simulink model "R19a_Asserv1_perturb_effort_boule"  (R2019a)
settings: Solver=ode15s  StartTime=0.0  StopTime=1  RelTol=1e-3  EnableMultiTasking=on
undefined symbols (not defined in the file): deg, kg, m, manette1_Défaut_sldprt, manette2_Défaut_sldprt, mm, N, rad, s, sigbuilder_block, STL, X, Y, Z
libraries: sm_lib x460, fl_lib x45, nesl_utility x23, simulink x3
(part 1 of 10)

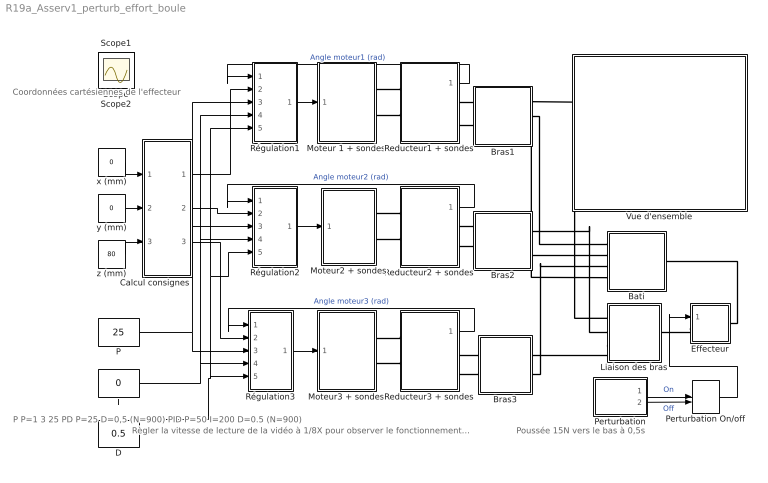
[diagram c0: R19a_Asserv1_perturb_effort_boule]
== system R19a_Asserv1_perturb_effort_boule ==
  note: P P=1 3 25 PD P=25 D=0,5 (N=900) PID P=50 I=200 D=0.5 (N=900)
  note: Coordonnées cartésiennes de l'effecteur
  note: Poussée 15N vers le bas à 0,5s
  note: Règler la vitesse de lecture de la vidéo à 1/8X pour observer le fonctionnement au ralenti
  Bati : Subsystem
  Bras1 : Subsystem
  Bras2 : Subsystem
  Bras3 : Subsystem
  Calcul consignes : Subsystem
  D : Constant  Value=0.5
  Effecteur : Subsystem
  I : Constant  Value=0
  Liaison des bras : Subsystem
  Moteur 1 + sondes : Subsystem
  Moteur2 + sondes : Subsystem
  Moteur3 + sondes : Subsystem
  P : Constant  Value=25
  Perturbation : Subsystem
  Perturbation On/off : ManualSwitch  CurrentSetting=0
  Reducteur1 + sondes : Subsystem
  Reducteur2 + sondes : Subsystem
  Reducteur3 + sondes : Subsystem
  Régulation1 : Subsystem
  Régulation2 : Subsystem
  Régulation3 : Subsystem
  Vue d'ensemble : Subsystem
  x (mm) : Constant  Value=0
  y (mm) : Constant  Value=0
  z (mm) : Constant  Value=80
  Scope : Scope
  Scope1 : Scope
  Scope2 : Scope
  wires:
  Régulation3/1(Out1) -> Moteur3 + sondes/1(In1)
  Reducteur3 + sondes/1(Angle_mot3) -> Régulation3/1(In1)  "Angle moteur3 (rad)"
  Régulation1/1(Out1) -> Moteur 1 + sondes/1(In1)
  Reducteur1 + sondes/1(Angle_mot1) -> Régulation1/1(In1)  "Angle moteur1 (rad)"
  Régulation2/1(Out1) -> Moteur2 + sondes/1(In1)
  Reducteur2 + sondes/1(Angle_mot2) -> Régulation2/1(In1)  "Angle moteur2 (rad)"
  Perturbation/1(Out1) -> Perturbation On/off/1  "On"
  Perturbation/2(Out2) -> Perturbation On/off/2  "Off"
  Perturbation On/off/1 -> Effecteur/1(In1)
  x (mm)/1 -> Calcul consignes/1(In1)
  y (mm)/1 -> Calcul consignes/2(In2)
  z (mm)/1 -> Calcul consignes/3(In3)
  Calcul consignes/1(C1) -> Régulation1/2(In2)
  Calcul consignes/2(C2) -> Régulation2/2(In2)
  Calcul consignes/3(C3) -> Régulation3/2(In2)
  P/1 -> Régulation3/3(P), Régulation1/3(P), Régulation2/3(P)
  I/1 -> Régulation1/4(I), Régulation2/4(I), Régulation3/4(I)
  D/1 -> Régulation1/5(D), Régulation2/5(D), Régulation3/5(D)
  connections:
  Moteur2 + sondes/RConn2 -- Reducteur2 + sondes/LConn2
  Moteur 1 + sondes/RConn1 -- Reducteur1 + sondes/LConn1
  Moteur3 + sondes/RConn2 -- Reducteur3 + sondes/LConn2
  Moteur2 + sondes/RConn1 -- Reducteur2 + sondes/LConn1
  Moteur3 + sondes/RConn1 -- Reducteur3 + sondes/LConn1
  Reducteur1 + sondes/LConn2 -- Moteur 1 + sondes/RConn2
  Bras1/LConn1 -- Reducteur1 + sondes/RConn1
  Reducteur1 + sondes/RConn2 -- Bras1/LConn2
  Bras2/LConn1 -- Reducteur2 + sondes/RConn1
  Bras2/LConn2 -- Reducteur2 + sondes/RConn2
  Reducteur3 + sondes/RConn1 -- Bras3/LConn1
  Reducteur3 + sondes/RConn2 -- Bras3/LConn2
  Bras1/RConn2 -- Bati/LConn1
  Bras2/RConn2 -- Bati/LConn2
  Bras3/RConn2 -- Bati/LConn3
  Liaison des bras/LConn1 -- Bras1/RConn1
  Liaison des bras/LConn2 -- Bras2/RConn1
  Effecteur/LConn1 -- Liaison des bras/RConn1
  Liaison des bras/LConn3 -- Bras3/RConn1
  Bati/RConn1 -- Effecteur/RConn1
  Bras1/RConn3 -- Bati/LConn4

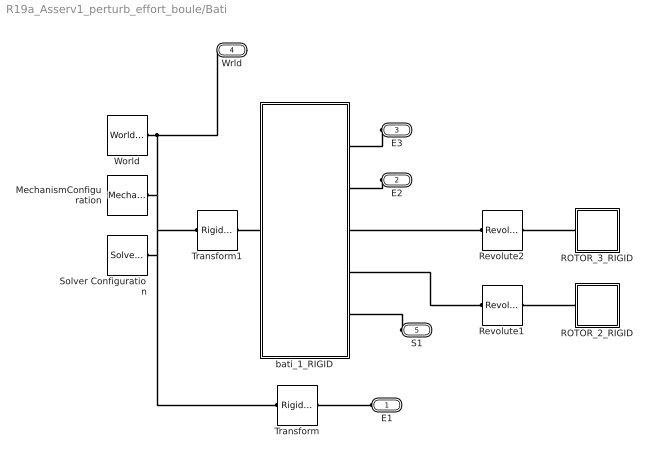
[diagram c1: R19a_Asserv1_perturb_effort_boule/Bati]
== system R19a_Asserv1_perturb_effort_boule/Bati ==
  MechanismConfiguration : sm_lib/Utilities/Mechanism Configuration  UniformGravity=Constant  GravityVector=[0 0 0]  GravityUnits=m/s^2  LinearizationDelta=0.001
  ROTOR_2_RIGID : Subsystem
  ROTOR_3_RIGID : Subsystem
  Revolute1 : sm_lib/Joints/Revolute Joint  SenseConstraintForce=off  SenseConstraintForceX=off  SenseConstraintForceY=off  SenseConstraintForceZ=off  SenseConstraintTorque=off  SenseConstraintTorqueX=off  SenseConstraintTorqueY=off  SenseConstraintTorqueZ=off  SenseTotalForce=off  SenseTotalForceX=off  SenseTotalForceY=off  SenseTotalForceZ=off  SenseTotalTorque=off  SenseTotalTorqueX=off  SenseTotalTorqueY=off  SenseTotalTorqueZ=off  CompositeWrenchDir=FollowerOnBase  CompositeWrenchFrame=BaseFrame  EquilibriumPosition=0  EquilibriumPositionUnits=rad  SpringStiffness=0  SpringStiffnessUnits=m*N/rad  DampingCoefficient=0  DampingCoefficientUnits=m*s*N/rad  TorqueActuationMode=NoTorque  MotionActuationMode=ComputedMotion  SensePosition=off  SenseVelocity=off  SenseAcceleration=off  SenseTorqueForce=off  SenseLowerLimitTorqueForce=off  SenseUpperLimitTorqueForce=off  LowerLimitSpecify=off  LowerLimitBound=-90  LowerLimitBoundUnits=deg  LowerLimitStiffness=1e4  LowerLimitStiffnessUnits=N*m/deg  LowerLimitDamping=10  LowerLimitDampingUnits=N*m/(deg/s)  LowerLimitTransitionRegionWidth=0.1  LowerLimitTransitionRegionWidthUnits=deg  UpperLimitSpecify=off  UpperLimitBound=90  UpperLimitBoundUnits=deg  UpperLimitStiffness=1e4  UpperLimitStiffnessUnits=N*m/deg  UpperLimitDamping=10  UpperLimitDampingUnits=N*m/(deg/s)  UpperLimitTransitionRegionWidth=0.1  UpperLimitTransitionRegionWidthUnits=deg  PositionTargetSpecify=on  PositionTargetPriority=Low  PositionTargetValue=-26.406351854743253  PositionTargetValueUnits=deg  VelocityTargetSpecify=off  VelocityTargetPriority=High  VelocityTargetValue=0  VelocityTargetValueUnits=deg/s
  Revolute2 : sm_lib/Joints/Revolute Joint  SenseConstraintForce=off  SenseConstraintForceX=off  SenseConstraintForceY=off  SenseConstraintForceZ=off  SenseConstraintTorque=off  SenseConstraintTorqueX=off  SenseConstraintTorqueY=off  SenseConstraintTorqueZ=off  SenseTotalForce=off  SenseTotalForceX=off  SenseTotalForceY=off  SenseTotalForceZ=off  SenseTotalTorque=off  SenseTotalTorqueX=off  SenseTotalTorqueY=off  SenseTotalTorqueZ=off  CompositeWrenchDir=FollowerOnBase  CompositeWrenchFrame=BaseFrame  EquilibriumPosition=0  EquilibriumPositionUnits=rad  SpringStiffness=0  SpringStiffnessUnits=m*N/rad  DampingCoefficient=0  DampingCoefficientUnits=m*s*N/rad  TorqueActuationMode=NoTorque  MotionActuationMode=ComputedMotion  SensePosition=off  SenseVelocity=off  SenseAcceleration=off  SenseTorqueForce=off  SenseLowerLimitTorqueForce=off  SenseUpperLimitTorqueForce=off  LowerLimitSpecify=off  LowerLimitBound=-90  LowerLimitBoundUnits=deg  LowerLimitStiffness=1e4  LowerLimitStiffnessUnits=N*m/deg  LowerLimitDamping=10  LowerLimitDampingUnits=N*m/(deg/s)  LowerLimitTransitionRegionWidth=0.1  LowerLimitTransitionRegionWidthUnits=deg  UpperLimitSpecify=off  UpperLimitBound=90  UpperLimitBoundUnits=deg  UpperLimitStiffness=1e4  UpperLimitStiffnessUnits=N*m/deg  UpperLimitDamping=10  UpperLimitDampingUnits=N*m/(deg/s)  UpperLimitTransitionRegionWidth=0.1  UpperLimitTransitionRegionWidthUnits=deg  PositionTargetSpecify=on  PositionTargetPriority=Low  PositionTargetValue=-61.713604489421797  PositionTargetValueUnits=deg  VelocityTargetSpecify=off  VelocityTargetPriority=High  VelocityTargetValue=0  VelocityTargetValueUnits=deg/s
  Solver Configuration : nesl_utility/Solver Configuration  PhysicalDomain=network_engine_domain  SubClassName=solver  LeftPortType=input  RightPortType=generic  Tones=[]  Harmonics=[]  SimulateNoise=off  Profile=off  UseLocalSampling=off  EnableSwitchedLinearOptims=on  FrequencyDomain=off  UseCCode=off  RelTol=0.001  AbsTol=1e-06  MinStep=1e-09  ToWorkspace=off  RevertToSquareIcSolve=off  NumHomotopyIterations=100  PhasorMode=off  PhasorModeNumHarmonics=1  DoDC=off  ResidualTolerance=1e-09  UseLocalSolver=off  LocalSolverChoice=NE_BACKWARD_EULER_ADVANCER  LocalSolverSampleTime=0.001  DoFixedCost=off  MaxNonlinIter=3  MaxModeIter=2  LinearAlgebra=Sparse  EquationFormulation=NE_TIME_EF  DelaysMemoryBudget=1024  AutomaticFiltering=on  FilteringTimeConstant=0.001  PartitionStorageMethod=AS_NEEDED  PartitionMemoryBudget=1024  PartitionMethod=FAST
  Transform : sm_lib/Frames and Transforms/Rigid Transform  TranslationMethod=Cartesian  TranslationStandardOffset=0  TranslationLengthUnit=mm  TranslationStandardAxis=+Z  TranslationCartesianOffset=[-50.295220189469383 24.641508789034031 0]  TranslationROffset=0  TranslationROffsetUnits=m  TranslationZOffset=0  TranslationZOffsetUnits=m  TranslationThetaOffset=0  TranslationThetaOffsetUnits=deg  RotationMethod=ArbitraryAxis  RotationAngleUnits=rad  RotationStandardAxis=+Z  RotationAngle=2.2576709855630148  RotationArbitraryAxis=[0.47317816576135285 0.62293756647304621 0.6229375664730461]  FollAlignAxisA=+X  BaseAlignAxisA=+Y  FollAlignAxisB=+Y  BaseAlignAxisB=+Z  RotationSequenceAxes=FollowerAxes  RotationSequence=XYX  RotationSequenceAngles=[0 0 0]  RotationSequenceAnglesUnits=deg  RotationMatrix=[1 0 0; 0 1 0; 0 0 1]
  Transform1 : sm_lib/Frames and Transforms/Rigid Transform  TranslationMethod=Cartesian  TranslationStandardOffset=0  TranslationLengthUnit=mm  TranslationStandardAxis=+Z  TranslationCartesianOffset=[0 -115.25004756062962 -99.318100969999989]  TranslationROffset=0  TranslationROffsetUnits=m  TranslationZOffset=0  TranslationZOffsetUnits=m  TranslationThetaOffset=0  TranslationThetaOffsetUnits=deg  RotationMethod=None  RotationAngleUnits=deg  RotationStandardAxis=+Z  RotationAngle=0  RotationArbitraryAxis=[0 0 1]  FollAlignAxisA=+X  BaseAlignAxisA=+Y  FollAlignAxisB=+Y  BaseAlignAxisB=+Z  RotationSequenceAxes=FollowerAxes  RotationSequence=XYX  RotationSequenceAngles=[0 0 0]  RotationSequenceAnglesUnits=deg  RotationMatrix=[1 0 0; 0 1 0; 0 0 1]
  World : sm_lib/Frames and Transforms/World Frame
  bati_1_RIGID : Subsystem
  E1 : PMIOPort  Side=Left
  E2 : PMIOPort  Port=2  Side=Left
  E3 : PMIOPort  Port=3  Side=Left
  Wrld : PMIOPort  Port=4  Side=Right
  S1 : PMIOPort  Port=5  Side=Left
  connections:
  MechanismConfiguration/RConn1 -- Transform/LConn1 -- Solver Configuration/RConn1 -- Transform1/LConn1 -- Wrld/RConn1 -- World/RConn1
  ROTOR_3_RIGID/LConn1 -- Revolute2/RConn1
  Transform1/RConn1 -- bati_1_RIGID/LConn1
  Revolute2/LConn1 -- bati_1_RIGID/RConn3
  E2/RConn1 -- bati_1_RIGID/RConn2
  E1/RConn1 -- Transform/RConn1
  E3/RConn1 -- bati_1_RIGID/RConn1
  ROTOR_2_RIGID/LConn1 -- Revolute1/RConn1
  S1/RConn1 -- bati_1_RIGID/RConn5
  Revolute1/LConn1 -- bati_1_RIGID/RConn4

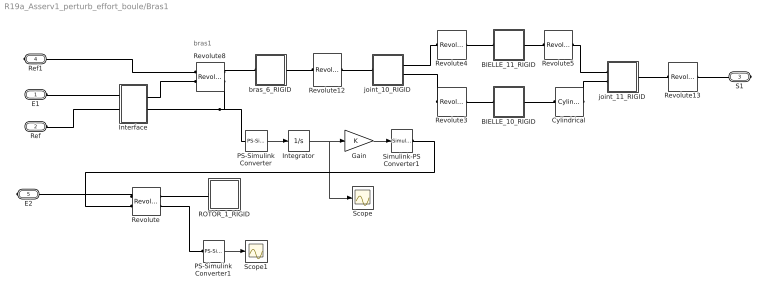
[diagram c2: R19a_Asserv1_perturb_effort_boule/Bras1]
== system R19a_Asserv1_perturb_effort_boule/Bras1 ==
  note: bras1
  BIELLE_10_RIGID : Subsystem
  BIELLE_11_RIGID : Subsystem
  Cylindrical : sm_lib/Joints/Cylindrical Joint  SenseConstraintForce=off  SenseConstraintForceX=off  SenseConstraintForceY=off  SenseConstraintForceZ=off  SenseConstraintTorque=off  SenseConstraintTorqueX=off  SenseConstraintTorqueY=off  SenseConstraintTorqueZ=off  SenseTotalForce=off  SenseTotalForceX=off  SenseTotalForceY=off  SenseTotalForceZ=off  SenseTotalTorque=off  SenseTotalTorqueX=off  SenseTotalTorqueY=off  SenseTotalTorqueZ=off  CompositeWrenchDir=FollowerOnBase  CompositeWrenchFrame=BaseFrame  PzEquilibriumPosition=0  PzEquilibriumPositionUnits=m  PzSpringStiffness=0  PzSpringStiffnessUnits=N/m  PzDampingCoefficient=0  PzDampingCoefficientUnits=s*N/m  PzTorqueActuationMode=NoTorque  PzMotionActuationMode=ComputedMotion  PzSensePosition=off  PzSenseVelocity=off  PzSenseAcceleration=off  PzSenseTorqueForce=off  PzSenseLowerLimitTorqueForce=off  PzSenseUpperLimitTorqueForce=off  PzLowerLimitSpecify=off  PzLowerLimitBound=-1  PzLowerLimitBoundUnits=m  PzLowerLimitStiffness=1e6  PzLowerLimitStiffnessUnits=N/m  PzLowerLimitDamping=1e3  PzLowerLimitDampingUnits=N/(m/s)  PzLowerLimitTransitionRegionWidth=1e-4  PzLowerLimitTransitionRegionWidthUnits=m  PzUpperLimitSpecify=off  PzUpperLimitBound=1  PzUpperLimitBoundUnits=m  PzUpperLimitStiffness=1e6  PzUpperLimitStiffnessUnits=N/m  PzUpperLimitDamping=1e3  PzUpperLimitDampingUnits=N/(m/s)  PzUpperLimitTransitionRegionWidth=1e-4  PzUpperLimitTransitionRegionWidthUnits=m  PzPositionTargetSpecify=off  PzPositionTargetPriority=High  PzPositionTargetValue=0  PzPositionTargetValueUnits=m  PzVelocityTargetSpecify=off  PzVelocityTargetPriority=High  PzVelocityTargetValue=0  PzVelocityTargetValueUnits=m/s  RzEquilibriumPosition=0  RzEquilibriumPositionUnits=rad  RzSpringStiffness=0  RzSpringStiffnessUnits=m*N/rad  RzDampingCoefficient=0  RzDampingCoefficientUnits=m*s*N/rad  RzTorqueActuationMode=NoTorque  RzMotionActuationMode=ComputedMotion  RzSensePosition=off  RzSenseVelocity=off  RzSenseAcceleration=off  RzSenseTorqueForce=off  RzSenseLowerLimitTorqueForce=off  RzSenseUpperLimitTorqueForce=off  RzLowerLimitSpecify=off  RzLowerLimitBound=-90  RzLowerLimitBoundUnits=deg  RzLowerLimitStiffness=1e4  RzLowerLimitStiffnessUnits=N*m/deg  RzLowerLimitDamping=10  RzLowerLimitDampingUnits=N*m/(deg/s)  RzLowerLimitTransitionRegionWidth=0.1  RzLowerLimitTransitionRegionWidthUnits=deg  RzUpperLimitSpecify=off  RzUpperLimitBound=90  RzUpperLimitBoundUnits=deg  RzUpperLimitStiffness=1e4  RzUpperLimitStiffnessUnits=N*m/deg  RzUpperLimitDamping=10  RzUpperLimitDampingUnits=N*m/(deg/s)  RzUpperLimitTransitionRegionWidth=0.1  RzUpperLimitTransitionRegionWidthUnits=deg  RzPositionTargetSpecify=off  RzPositionTargetPriority=High  RzPositionTargetValue=0  RzPositionTargetValueUnits=deg  RzVelocityTargetSpecify=off  RzVelocityTargetPriority=High  RzVelocityTargetValue=0  RzVelocityTargetValueUnits=deg/s
  Gain : Gain
  Integrator : Integrator
  Interface : Subsystem
  PS-Simulink Converter : nesl_utility/PS-Simulink Converter  PhysicalDomain=network_engine_domain  SubClassName=ps_output  LeftPortType=input  RightPortType=output  PseudoPeriodic=off  Frequencies=[]  Unit=1  AffineConversion=off
  PS-Simulink Converter1 : nesl_utility/PS-Simulink Converter  PhysicalDomain=network_engine_domain  SubClassName=ps_output  LeftPortType=input  RightPortType=output  PseudoPeriodic=off  Frequencies=[]  Unit=1  AffineConversion=off
  ROTOR_1_RIGID : Subsystem
  Revolute : sm_lib/Joints/Revolute Joint  SenseConstraintForce=off  SenseConstraintForceX=off  SenseConstraintForceY=off  SenseConstraintForceZ=off  SenseConstraintTorque=off  SenseConstraintTorqueX=off  SenseConstraintTorqueY=off  SenseConstraintTorqueZ=off  SenseTotalForce=off  SenseTotalForceX=off  SenseTotalForceY=off  SenseTotalForceZ=off  SenseTotalTorque=off  SenseTotalTorqueX=off  SenseTotalTorqueY=off  SenseTotalTorqueZ=off  CompositeWrenchDir=FollowerOnBase  CompositeWrenchFrame=BaseFrame  EquilibriumPosition=0  EquilibriumPositionUnits=rad  SpringStiffness=0  SpringStiffnessUnits=m*N/rad  DampingCoefficient=0  DampingCoefficientUnits=m*s*N/rad  TorqueActuationMode=ComputedTorque  MotionActuationMode=InputMotion  SensePosition=off  SenseVelocity=on  SenseAcceleration=off  SenseTorqueForce=off  SenseLowerLimitTorqueForce=off  SenseUpperLimitTorqueForce=off  LowerLimitSpecify=off  LowerLimitBound=-90  LowerLimitBoundUnits=deg  LowerLimitStiffness=1e4  LowerLimitStiffnessUnits=N*m/deg  LowerLimitDamping=10  LowerLimitDampingUnits=N*m/(deg/s)  LowerLimitTransitionRegionWidth=0.1  LowerLimitTransitionRegionWidthUnits=deg  UpperLimitSpecify=off  UpperLimitBound=90  UpperLimitBoundUnits=deg  UpperLimitStiffness=1e4  UpperLimitStiffnessUnits=N*m/deg  UpperLimitDamping=10  UpperLimitDampingUnits=N*m/(deg/s)  UpperLimitTransitionRegionWidth=0.1  UpperLimitTransitionRegionWidthUnits=deg  PositionTargetSpecify=on  PositionTargetPriority=Low  PositionTargetValue=-79.560971310790379  PositionTargetValueUnits=deg  VelocityTargetSpecify=off  VelocityTargetPriority=High  VelocityTargetValue=0  VelocityTargetValueUnits=deg/s
  Revolute12 : sm_lib/Joints/Revolute Joint  SenseConstraintForce=off  SenseConstraintForceX=off  SenseConstraintForceY=off  SenseConstraintForceZ=off  SenseConstraintTorque=off  SenseConstraintTorqueX=off  SenseConstraintTorqueY=off  SenseConstraintTorqueZ=off  SenseTotalForce=off  SenseTotalForceX=off  SenseTotalForceY=off  SenseTotalForceZ=off  SenseTotalTorque=off  SenseTotalTorqueX=off  SenseTotalTorqueY=off  SenseTotalTorqueZ=off  CompositeWrenchDir=FollowerOnBase  CompositeWrenchFrame=BaseFrame  EquilibriumPosition=0  EquilibriumPositionUnits=rad  SpringStiffness=0  SpringStiffnessUnits=m*N/rad  DampingCoefficient=0  DampingCoefficientUnits=m*s*N/rad  TorqueActuationMode=NoTorque  MotionActuationMode=ComputedMotion  SensePosition=off  SenseVelocity=off  SenseAcceleration=off  SenseTorqueForce=off  SenseLowerLimitTorqueForce=off  SenseUpperLimitTorqueForce=off  LowerLimitSpecify=off  LowerLimitBound=-90  LowerLimitBoundUnits=deg  LowerLimitStiffness=1e4  LowerLimitStiffnessUnits=N*m/deg  LowerLimitDamping=10  LowerLimitDampingUnits=N*m/(deg/s)  LowerLimitTransitionRegionWidth=0.1  LowerLimitTransitionRegionWidthUnits=deg  UpperLimitSpecify=off  UpperLimitBound=90  UpperLimitBoundUnits=deg  UpperLimitStiffness=1e4  UpperLimitStiffnessUnits=N*m/deg  UpperLimitDamping=10  UpperLimitDampingUnits=N*m/(deg/s)  UpperLimitTransitionRegionWidth=0.1  UpperLimitTransitionRegionWidthUnits=deg  PositionTargetSpecify=on  PositionTargetPriority=Low  PositionTargetValue=114.87234196171698  PositionTargetValueUnits=deg  VelocityTargetSpecify=off  VelocityTargetPriority=High  VelocityTargetValue=0  VelocityTargetValueUnits=deg/s
  Revolute13 : sm_lib/Joints/Revolute Joint  SenseConstraintForce=off  SenseConstraintForceX=off  SenseConstraintForceY=off  SenseConstraintForceZ=off  SenseConstraintTorque=off  SenseConstraintTorqueX=off  SenseConstraintTorqueY=off  SenseConstraintTorqueZ=off  SenseTotalForce=off  SenseTotalForceX=off  SenseTotalForceY=off  SenseTotalForceZ=off  SenseTotalTorque=off  SenseTotalTorqueX=off  SenseTotalTorqueY=off  SenseTotalTorqueZ=off  CompositeWrenchDir=FollowerOnBase  CompositeWrenchFrame=BaseFrame  EquilibriumPosition=0  EquilibriumPositionUnits=rad  SpringStiffness=0  SpringStiffnessUnits=m*N/rad  DampingCoefficient=0  DampingCoefficientUnits=m*s*N/rad  TorqueActuationMode=NoTorque  MotionActuationMode=ComputedMotion  SensePosition=off  SenseVelocity=off  SenseAcceleration=off  SenseTorqueForce=off  SenseLowerLimitTorqueForce=off  SenseUpperLimitTorqueForce=off  LowerLimitSpecify=off  LowerLimitBound=-90  LowerLimitBoundUnits=deg  LowerLimitStiffness=1e4  LowerLimitStiffnessUnits=N*m/deg  LowerLimitDamping=10  LowerLimitDampingUnits=N*m/(deg/s)  LowerLimitTransitionRegionWidth=0.1  LowerLimitTransitionRegionWidthUnits=deg  UpperLimitSpecify=off  UpperLimitBound=90  UpperLimitBoundUnits=deg  UpperLimitStiffness=1e4  UpperLimitStiffnessUnits=N*m/deg  UpperLimitDamping=10  UpperLimitDampingUnits=N*m/(deg/s)  UpperLimitTransitionRegionWidth=0.1  UpperLimitTransitionRegionWidthUnits=deg  PositionTargetSpecify=off  PositionTargetPriority=High  PositionTargetValue=0  PositionTargetValueUnits=deg  VelocityTargetSpecify=off  VelocityTargetPriority=High  VelocityTargetValue=0  VelocityTargetValueUnits=deg/s
  Revolute3 : sm_lib/Joints/Revolute Joint  SenseConstraintForce=off  SenseConstraintForceX=off  SenseConstraintForceY=off  SenseConstraintForceZ=off  SenseConstraintTorque=off  SenseConstraintTorqueX=off  SenseConstraintTorqueY=off  SenseConstraintTorqueZ=off  SenseTotalForce=off  SenseTotalForceX=off  SenseTotalForceY=off  SenseTotalForceZ=off  SenseTotalTorque=off  SenseTotalTorqueX=off  SenseTotalTorqueY=off  SenseTotalTorqueZ=off  CompositeWrenchDir=FollowerOnBase  CompositeWrenchFrame=BaseFrame  EquilibriumPosition=0  EquilibriumPositionUnits=rad  SpringStiffness=0  SpringStiffnessUnits=m*N/rad  DampingCoefficient=0  DampingCoefficientUnits=m*s*N/rad  TorqueActuationMode=NoTorque  MotionActuationMode=ComputedMotion  SensePosition=off  SenseVelocity=off  SenseAcceleration=off  SenseTorqueForce=off  SenseLowerLimitTorqueForce=off  SenseUpperLimitTorqueForce=off  LowerLimitSpecify=off  LowerLimitBound=-90  LowerLimitBoundUnits=deg  LowerLimitStiffness=1e4  LowerLimitStiffnessUnits=N*m/deg  LowerLimitDamping=10  LowerLimitDampingUnits=N*m/(deg/s)  LowerLimitTransitionRegionWidth=0.1  LowerLimitTransitionRegionWidthUnits=deg  UpperLimitSpecify=off  UpperLimitBound=90  UpperLimitBoundUnits=deg  UpperLimitStiffness=1e4  UpperLimitStiffnessUnits=N*m/deg  UpperLimitDamping=10  UpperLimitDampingUnits=N*m/(deg/s)  UpperLimitTransitionRegionWidth=0.1  UpperLimitTransitionRegionWidthUnits=deg  PositionTargetSpecify=on  PositionTargetPriority=Low  PositionTargetValue=-1.4448284825041595  PositionTargetValueUnits=deg  VelocityTargetSpecify=off  VelocityTargetPriority=High  VelocityTargetValue=0  VelocityTargetValueUnits=deg/s
  Revolute4 : sm_lib/Joints/Revolute Joint  SenseConstraintForce=off  SenseConstraintForceX=off  SenseConstraintForceY=off  SenseConstraintForceZ=off  SenseConstraintTorque=off  SenseConstraintTorqueX=off  SenseConstraintTorqueY=off  SenseConstraintTorqueZ=off  SenseTotalForce=off  SenseTotalForceX=off  SenseTotalForceY=off  SenseTotalForceZ=off  SenseTotalTorque=off  SenseTotalTorqueX=off  SenseTotalTorqueY=off  SenseTotalTorqueZ=off  CompositeWrenchDir=FollowerOnBase  CompositeWrenchFrame=BaseFrame  EquilibriumPosition=0  EquilibriumPositionUnits=rad  SpringStiffness=0  SpringStiffnessUnits=m*N/rad  DampingCoefficient=0  DampingCoefficientUnits=m*s*N/rad  TorqueActuationMode=NoTorque  MotionActuationMode=ComputedMotion  SensePosition=off  SenseVelocity=off  SenseAcceleration=off  SenseTorqueForce=off  SenseLowerLimitTorqueForce=off  SenseUpperLimitTorqueForce=off  LowerLimitSpecify=off  LowerLimitBound=-90  LowerLimitBoundUnits=deg  LowerLimitStiffness=1e4  LowerLimitStiffnessUnits=N*m/deg  LowerLimitDamping=10  LowerLimitDampingUnits=N*m/(deg/s)  LowerLimitTransitionRegionWidth=0.1  LowerLimitTransitionRegionWidthUnits=deg  UpperLimitSpecify=off  UpperLimitBound=90  UpperLimitBoundUnits=deg  UpperLimitStiffness=1e4  UpperLimitStiffnessUnits=N*m/deg  UpperLimitDamping=10  UpperLimitDampingUnits=N*m/(deg/s)  UpperLimitTransitionRegionWidth=0.1  UpperLimitTransitionRegionWidthUnits=deg  PositionTargetSpecify=on  PositionTargetPriority=Low  PositionTargetValue=1.4448284825041535  PositionTargetValueUnits=deg  VelocityTargetSpecify=off  VelocityTargetPriority=High  VelocityTargetValue=0  VelocityTargetValueUnits=deg/s
  Revolute5 : sm_lib/Joints/Revolute Joint  SenseConstraintForce=off  SenseConstraintForceX=off  SenseConstraintForceY=off  SenseConstraintForceZ=off  SenseConstraintTorque=off  SenseConstraintTorqueX=off  SenseConstraintTorqueY=off  SenseConstraintTorqueZ=off  SenseTotalForce=off  SenseTotalForceX=off  SenseTotalForceY=off  SenseTotalForceZ=off  SenseTotalTorque=off  SenseTotalTorqueX=off  SenseTotalTorqueY=off  SenseTotalTorqueZ=off  CompositeWrenchDir=FollowerOnBase  CompositeWrenchFrame=BaseFrame  EquilibriumPosition=0  EquilibriumPositionUnits=rad  SpringStiffness=0  SpringStiffnessUnits=m*N/rad  DampingCoefficient=0  DampingCoefficientUnits=m*s*N/rad  TorqueActuationMode=NoTorque  MotionActuationMode=ComputedMotion  SensePosition=off  SenseVelocity=off  SenseAcceleration=off  SenseTorqueForce=off  SenseLowerLimitTorqueForce=off  SenseUpperLimitTorqueForce=off  LowerLimitSpecify=off  LowerLimitBound=-90  LowerLimitBoundUnits=deg  LowerLimitStiffness=1e4  LowerLimitStiffnessUnits=N*m/deg  LowerLimitDamping=10  LowerLimitDampingUnits=N*m/(deg/s)  LowerLimitTransitionRegionWidth=0.1  LowerLimitTransitionRegionWidthUnits=deg  UpperLimitSpecify=off  UpperLimitBound=90  UpperLimitBoundUnits=deg  UpperLimitStiffness=1e4  UpperLimitStiffnessUnits=N*m/deg  UpperLimitDamping=10  UpperLimitDampingUnits=N*m/(deg/s)  UpperLimitTransitionRegionWidth=0.1  UpperLimitTransitionRegionWidthUnits=deg  PositionTargetSpecify=on  PositionTargetPriority=Low  PositionTargetValue=-178.55517151749589  PositionTargetValueUnits=deg  VelocityTargetSpecify=off  VelocityTargetPriority=High  VelocityTargetValue=0  VelocityTargetValueUnits=deg/s
  Revolute8 : sm_lib/Joints/Revolute Joint  SenseConstraintForce=off  SenseConstraintForceX=off  SenseConstraintForceY=off  SenseConstraintForceZ=off  SenseConstraintTorque=off  SenseConstraintTorqueX=off  SenseConstraintTorqueY=off  SenseConstraintTorqueZ=off  SenseTotalForce=off  SenseTotalForceX=off  SenseTotalForceY=off  SenseTotalForceZ=off  SenseTotalTorque=off  SenseTotalTorqueX=off  SenseTotalTorqueY=off  SenseTotalTorqueZ=off  CompositeWrenchDir=FollowerOnBase  CompositeWrenchFrame=BaseFrame  EquilibriumPosition=0  EquilibriumPositionUnits=rad  SpringStiffness=0  SpringStiffnessUnits=m*N/rad  DampingCoefficient=0  DampingCoefficientUnits=m*s*N/rad  TorqueActuationMode=InputTorque  MotionActuationMode=ComputedMotion  SensePosition=off  SenseVelocity=on  SenseAcceleration=off  SenseTorqueForce=off  SenseLowerLimitTorqueForce=off  SenseUpperLimitTorqueForce=off  LowerLimitSpecify=off  LowerLimitBound=-90  LowerLimitBoundUnits=deg  LowerLimitStiffness=1e4  LowerLimitStiffnessUnits=N*m/deg  LowerLimitDamping=10  LowerLimitDampingUnits=N*m/(deg/s)  LowerLimitTransitionRegionWidth=0.1  LowerLimitTransitionRegionWidthUnits=deg  UpperLimitSpecify=off  UpperLimitBound=90  UpperLimitBoundUnits=deg  UpperLimitStiffness=1e4  UpperLimitStiffnessUnits=N*m/deg  UpperLimitDamping=10  UpperLimitDampingUnits=N*m/(deg/s)  UpperLimitTransitionRegionWidth=0.1  UpperLimitTransitionRegionWidthUnits=deg  PositionTargetSpecify=on  PositionTargetPriority=Low  PositionTargetValue=-11.877849818911594  PositionTargetValueUnits=deg  VelocityTargetSpecify=off  VelocityTargetPriority=High  VelocityTargetValue=0  VelocityTargetValueUnits=deg/s
  Scope : Scope
  Scope1 : Scope
  Simulink-PS Converter1 : nesl_utility/Simulink-PS Converter  PhysicalDomain=network_engine_domain  SubClassName=ps_input  LeftPortType=input  RightPortType=output  PseudoPeriodic=off  Frequencies=[]  NoiseDistribution=none  NoiseParameters=[]  Unit=1  AffineConversion=off  FilteringAndDerivatives=filter  SimscapeFilterOrder=2  InputFilterTimeConstant=1e-4  UdotUserProvided=1
  bras_6_RIGID : Subsystem
  joint_10_RIGID : Subsystem
  joint_11_RIGID : Subsystem
  E1 : PMIOPort  Side=Left
  Ref : PMIOPort  Port=2  Side=Left
  S1 : PMIOPort  Port=3  Side=Right
  Ref1 : PMIOPort  Port=4  Side=Right
  E2 : PMIOPort  Port=5  Side=Right
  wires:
  PS-Simulink Converter/1 -> Integrator/1
  Gain/1 -> Simulink-PS Converter1/1
  PS-Simulink Converter1/1 -> Scope1/1
  Integrator/1 -> Scope/1, Gain/1
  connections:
  Interface/RConn1 -- Revolute8/LConn2
  Interface/RConn2 -- PS-Simulink Converter/LConn1 -- Revolute8/RConn2
  Ref/RConn1 -- Interface/LConn2
  Interface/LConn1 -- E1/RConn1
  BIELLE_11_RIGID/LConn1 -- Revolute4/LConn1
  BIELLE_10_RIGID/RConn1 -- Cylindrical/LConn1
  Revolute4/RConn1 -- joint_10_RIGID/RConn1
  Cylindrical/RConn1 -- joint_11_RIGID/LConn2
  BIELLE_11_RIGID/RConn1 -- Revolute5/LConn1
  Revolute12/LConn1 -- bras_6_RIGID/RConn1
  Revolute12/RConn1 -- joint_10_RIGID/LConn1
  Revolute8/RConn1 -- bras_6_RIGID/LConn1
  Revolute8/LConn1 -- Ref1/RConn1
  Revolute5/RConn1 -- joint_11_RIGID/LConn1
  Revolute13/RConn1 -- joint_11_RIGID/RConn1
  S1/RConn1 -- Revolute13/LConn1
  Revolute3/RConn1 -- joint_10_RIGID/RConn2
  BIELLE_10_RIGID/LConn1 -- Revolute3/LConn1
  ROTOR_1_RIGID/LConn1 -- Revolute/RConn1
  Revolute/LConn1 -- E2/RConn1
  Revolute/LConn2 -- Simulink-PS Converter1/RConn1
  PS-Simulink Converter1/LConn1 -- Revolute/RConn2

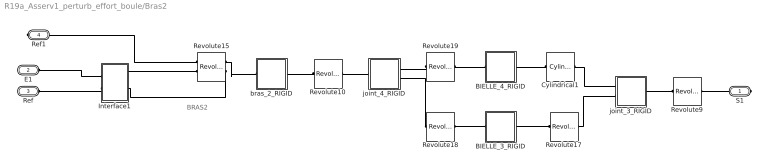
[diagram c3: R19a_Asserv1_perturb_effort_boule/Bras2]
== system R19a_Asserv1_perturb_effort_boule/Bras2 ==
  note: BRAS2
  BIELLE_3_RIGID : Subsystem
  BIELLE_4_RIGID : Subsystem
  Cylindrical1 : sm_lib/Joints/Cylindrical Joint  SenseConstraintForce=off  SenseConstraintForceX=off  SenseConstraintForceY=off  SenseConstraintForceZ=off  SenseConstraintTorque=off  SenseConstraintTorqueX=off  SenseConstraintTorqueY=off  SenseConstraintTorqueZ=off  SenseTotalForce=off  SenseTotalForceX=off  SenseTotalForceY=off  SenseTotalForceZ=off  SenseTotalTorque=off  SenseTotalTorqueX=off  SenseTotalTorqueY=off  SenseTotalTorqueZ=off  CompositeWrenchDir=FollowerOnBase  CompositeWrenchFrame=BaseFrame  PzEquilibriumPosition=0  PzEquilibriumPositionUnits=m  PzSpringStiffness=0  PzSpringStiffnessUnits=N/m  PzDampingCoefficient=0  PzDampingCoefficientUnits=s*N/m  PzTorqueActuationMode=NoTorque  PzMotionActuationMode=ComputedMotion  PzSensePosition=off  PzSenseVelocity=off  PzSenseAcceleration=off  PzSenseTorqueForce=off  PzSenseLowerLimitTorqueForce=off  PzSenseUpperLimitTorqueForce=off  PzLowerLimitSpecify=off  PzLowerLimitBound=-1  PzLowerLimitBoundUnits=m  PzLowerLimitStiffness=1e6  PzLowerLimitStiffnessUnits=N/m  PzLowerLimitDamping=1e3  PzLowerLimitDampingUnits=N/(m/s)  PzLowerLimitTransitionRegionWidth=1e-4  PzLowerLimitTransitionRegionWidthUnits=m  PzUpperLimitSpecify=off  PzUpperLimitBound=1  PzUpperLimitBoundUnits=m  PzUpperLimitStiffness=1e6  PzUpperLimitStiffnessUnits=N/m  PzUpperLimitDamping=1e3  PzUpperLimitDampingUnits=N/(m/s)  PzUpperLimitTransitionRegionWidth=1e-4  PzUpperLimitTransitionRegionWidthUnits=m  PzPositionTargetSpecify=off  PzPositionTargetPriority=High  PzPositionTargetValue=0  PzPositionTargetValueUnits=m  PzVelocityTargetSpecify=off  PzVelocityTargetPriority=High  PzVelocityTargetValue=0  PzVelocityTargetValueUnits=m/s  RzEquilibriumPosition=0  RzEquilibriumPositionUnits=rad  RzSpringStiffness=0  RzSpringStiffnessUnits=m*N/rad  RzDampingCoefficient=0  RzDampingCoefficientUnits=m*s*N/rad  RzTorqueActuationMode=NoTorque  RzMotionActuationMode=ComputedMotion  RzSensePosition=off  RzSenseVelocity=off  RzSenseAcceleration=off  RzSenseTorqueForce=off  RzSenseLowerLimitTorqueForce=off  RzSenseUpperLimitTorqueForce=off  RzLowerLimitSpecify=off  RzLowerLimitBound=-90  RzLowerLimitBoundUnits=deg  RzLowerLimitStiffness=1e4  RzLowerLimitStiffnessUnits=N*m/deg  RzLowerLimitDamping=10  RzLowerLimitDampingUnits=N*m/(deg/s)  RzLowerLimitTransitionRegionWidth=0.1  RzLowerLimitTransitionRegionWidthUnits=deg  RzUpperLimitSpecify=off  RzUpperLimitBound=90  RzUpperLimitBoundUnits=deg  RzUpperLimitStiffness=1e4  RzUpperLimitStiffnessUnits=N*m/deg  RzUpperLimitDamping=10  RzUpperLimitDampingUnits=N*m/(deg/s)  RzUpperLimitTransitionRegionWidth=0.1  RzUpperLimitTransitionRegionWidthUnits=deg  RzPositionTargetSpecify=off  RzPositionTargetPriority=High  RzPositionTargetValue=0  RzPositionTargetValueUnits=deg  RzVelocityTargetSpecify=off  RzVelocityTargetPriority=High  RzVelocityTargetValue=0  RzVelocityTargetValueUnits=deg/s
  Interface1 : Subsystem
  Revolute10 : sm_lib/Joints/Revolute Joint  SenseConstraintForce=off  SenseConstraintForceX=off  SenseConstraintForceY=off  SenseConstraintForceZ=off  SenseConstraintTorque=off  SenseConstraintTorqueX=off  SenseConstraintTorqueY=off  SenseConstraintTorqueZ=off  SenseTotalForce=off  SenseTotalForceX=off  SenseTotalForceY=off  SenseTotalForceZ=off  SenseTotalTorque=off  SenseTotalTorqueX=off  SenseTotalTorqueY=off  SenseTotalTorqueZ=off  CompositeWrenchDir=FollowerOnBase  CompositeWrenchFrame=BaseFrame  EquilibriumPosition=0  EquilibriumPositionUnits=rad  SpringStiffness=0  SpringStiffnessUnits=m*N/rad  DampingCoefficient=0  DampingCoefficientUnits=m*s*N/rad  TorqueActuationMode=NoTorque  MotionActuationMode=ComputedMotion  SensePosition=off  SenseVelocity=off  SenseAcceleration=off  SenseTorqueForce=off  SenseLowerLimitTorqueForce=off  SenseUpperLimitTorqueForce=off  LowerLimitSpecify=off  LowerLimitBound=-90  LowerLimitBoundUnits=deg  LowerLimitStiffness=1e4  LowerLimitStiffnessUnits=N*m/deg  LowerLimitDamping=10  LowerLimitDampingUnits=N*m/(deg/s)  LowerLimitTransitionRegionWidth=0.1  LowerLimitTransitionRegionWidthUnits=deg  UpperLimitSpecify=off  UpperLimitBound=90  UpperLimitBoundUnits=deg  UpperLimitStiffness=1e4  UpperLimitStiffnessUnits=N*m/deg  UpperLimitDamping=10  UpperLimitDampingUnits=N*m/(deg/s)  UpperLimitTransitionRegionWidth=0.1  UpperLimitTransitionRegionWidthUnits=deg  PositionTargetSpecify=on  PositionTargetPriority=Low  PositionTargetValue=114.872364906431  PositionTargetValueUnits=deg  VelocityTargetSpecify=off  VelocityTargetPriority=High  VelocityTargetValue=0  VelocityTargetValueUnits=deg/s
  Revolute15 : sm_lib/Joints/Revolute Joint  SenseConstraintForce=off  SenseConstraintForceX=off  SenseConstraintForceY=off  SenseConstraintForceZ=off  SenseConstraintTorque=off  SenseConstraintTorqueX=off  SenseConstraintTorqueY=off  SenseConstraintTorqueZ=off  SenseTotalForce=off  SenseTotalForceX=off  SenseTotalForceY=off  SenseTotalForceZ=off  SenseTotalTorque=off  SenseTotalTorqueX=off  SenseTotalTorqueY=off  SenseTotalTorqueZ=off  CompositeWrenchDir=FollowerOnBase  CompositeWrenchFrame=BaseFrame  EquilibriumPosition=0  EquilibriumPositionUnits=rad  SpringStiffness=0  SpringStiffnessUnits=m*N/rad  DampingCoefficient=0  DampingCoefficientUnits=m*s*N/rad  TorqueActuationMode=InputTorque  MotionActuationMode=ComputedMotion  SensePosition=off  SenseVelocity=on  SenseAcceleration=off  SenseTorqueForce=off  SenseLowerLimitTorqueForce=off  SenseUpperLimitTorqueForce=off  LowerLimitSpecify=off  LowerLimitBound=-90  LowerLimitBoundUnits=deg  LowerLimitStiffness=1e4  LowerLimitStiffnessUnits=N*m/deg  LowerLimitDamping=10  LowerLimitDampingUnits=N*m/(deg/s)  LowerLimitTransitionRegionWidth=0.1  LowerLimitTransitionRegionWidthUnits=deg  UpperLimitSpecify=off  UpperLimitBound=90  UpperLimitBoundUnits=deg  UpperLimitStiffness=1e4  UpperLimitStiffnessUnits=N*m/deg  UpperLimitDamping=10  UpperLimitDampingUnits=N*m/(deg/s)  UpperLimitTransitionRegionWidth=0.1  UpperLimitTransitionRegionWidthUnits=deg  PositionTargetSpecify=on  PositionTargetPriority=Low  PositionTargetValue=-168.12223208512529  PositionTargetValueUnits=deg  VelocityTargetSpecify=off  VelocityTargetPriority=High  VelocityTargetValue=0  VelocityTargetValueUnits=deg/s
  Revolute17 : sm_lib/Joints/Revolute Joint  SenseConstraintForce=off  SenseConstraintForceX=off  SenseConstraintForceY=off  SenseConstraintForceZ=off  SenseConstraintTorque=off  SenseConstraintTorqueX=off  SenseConstraintTorqueY=off  SenseConstraintTorqueZ=off  SenseTotalForce=off  SenseTotalForceX=off  SenseTotalForceY=off  SenseTotalForceZ=off  SenseTotalTorque=off  SenseTotalTorqueX=off  SenseTotalTorqueY=off  SenseTotalTorqueZ=off  CompositeWrenchDir=FollowerOnBase  CompositeWrenchFrame=BaseFrame  EquilibriumPosition=0  EquilibriumPositionUnits=rad  SpringStiffness=0  SpringStiffnessUnits=m*N/rad  DampingCoefficient=0  DampingCoefficientUnits=m*s*N/rad  TorqueActuationMode=NoTorque  MotionActuationMode=ComputedMotion  SensePosition=off  SenseVelocity=off  SenseAcceleration=off  SenseTorqueForce=off  SenseLowerLimitTorqueForce=off  SenseUpperLimitTorqueForce=off  LowerLimitSpecify=off  LowerLimitBound=-90  LowerLimitBoundUnits=deg  LowerLimitStiffness=1e4  LowerLimitStiffnessUnits=N*m/deg  LowerLimitDamping=10  LowerLimitDampingUnits=N*m/(deg/s)  LowerLimitTransitionRegionWidth=0.1  LowerLimitTransitionRegionWidthUnits=deg  UpperLimitSpecify=off  UpperLimitBound=90  UpperLimitBoundUnits=deg  UpperLimitStiffness=1e4  UpperLimitStiffnessUnits=N*m/deg  UpperLimitDamping=10  UpperLimitDampingUnits=N*m/(deg/s)  UpperLimitTransitionRegionWidth=0.1  UpperLimitTransitionRegionWidthUnits=deg  PositionTargetSpecify=on  PositionTargetPriority=Low  PositionTargetValue=-1.4448169961462776  PositionTargetValueUnits=deg  VelocityTargetSpecify=off  VelocityTargetPriority=High  VelocityTargetValue=0  VelocityTargetValueUnits=deg/s
  Revolute18 : sm_lib/Joints/Revolute Joint  SenseConstraintForce=off  SenseConstraintForceX=off  SenseConstraintForceY=off  SenseConstraintForceZ=off  SenseConstraintTorque=off  SenseConstraintTorqueX=off  SenseConstraintTorqueY=off  SenseConstraintTorqueZ=off  SenseTotalForce=off  SenseTotalForceX=off  SenseTotalForceY=off  SenseTotalForceZ=off  SenseTotalTorque=off  SenseTotalTorqueX=off  SenseTotalTorqueY=off  SenseTotalTorqueZ=off  CompositeWrenchDir=FollowerOnBase  CompositeWrenchFrame=BaseFrame  EquilibriumPosition=0  EquilibriumPositionUnits=rad  SpringStiffness=0  SpringStiffnessUnits=m*N/rad  DampingCoefficient=0  DampingCoefficientUnits=m*s*N/rad  TorqueActuationMode=NoTorque  MotionActuationMode=ComputedMotion  SensePosition=off  SenseVelocity=off  SenseAcceleration=off  SenseTorqueForce=off  SenseLowerLimitTorqueForce=off  SenseUpperLimitTorqueForce=off  LowerLimitSpecify=off  LowerLimitBound=-90  LowerLimitBoundUnits=deg  LowerLimitStiffness=1e4  LowerLimitStiffnessUnits=N*m/deg  LowerLimitDamping=10  LowerLimitDampingUnits=N*m/(deg/s)  LowerLimitTransitionRegionWidth=0.1  LowerLimitTransitionRegionWidthUnits=deg  UpperLimitSpecify=off  UpperLimitBound=90  UpperLimitBoundUnits=deg  UpperLimitStiffness=1e4  UpperLimitStiffnessUnits=N*m/deg  UpperLimitDamping=10  UpperLimitDampingUnits=N*m/(deg/s)  UpperLimitTransitionRegionWidth=0.1  UpperLimitTransitionRegionWidthUnits=deg  PositionTargetSpecify=on  PositionTargetPriority=Low  PositionTargetValue=178.55518300385469  PositionTargetValueUnits=deg  VelocityTargetSpecify=off  VelocityTargetPriority=High  VelocityTargetValue=0  VelocityTargetValueUnits=deg/s
  Revolute19 : sm_lib/Joints/Revolute Joint  SenseConstraintForce=off  SenseConstraintForceX=off  SenseConstraintForceY=off  SenseConstraintForceZ=off  SenseConstraintTorque=off  SenseConstraintTorqueX=off  SenseConstraintTorqueY=off  SenseConstraintTorqueZ=off  SenseTotalForce=off  SenseTotalForceX=off  SenseTotalForceY=off  SenseTotalForceZ=off  SenseTotalTorque=off  SenseTotalTorqueX=off  SenseTotalTorqueY=off  SenseTotalTorqueZ=off  CompositeWrenchDir=FollowerOnBase  CompositeWrenchFrame=BaseFrame  EquilibriumPosition=0  EquilibriumPositionUnits=rad  SpringStiffness=0  SpringStiffnessUnits=m*N/rad  DampingCoefficient=0  DampingCoefficientUnits=m*s*N/rad  TorqueActuationMode=NoTorque  MotionActuationMode=ComputedMotion  SensePosition=off  SenseVelocity=off  SenseAcceleration=off  SenseTorqueForce=off  SenseLowerLimitTorqueForce=off  SenseUpperLimitTorqueForce=off  LowerLimitSpecify=off  LowerLimitBound=-90  LowerLimitBoundUnits=deg  LowerLimitStiffness=1e4  LowerLimitStiffnessUnits=N*m/deg  LowerLimitDamping=10  LowerLimitDampingUnits=N*m/(deg/s)  LowerLimitTransitionRegionWidth=0.1  LowerLimitTransitionRegionWidthUnits=deg  UpperLimitSpecify=off  UpperLimitBound=90  UpperLimitBoundUnits=deg  UpperLimitStiffness=1e4  UpperLimitStiffnessUnits=N*m/deg  UpperLimitDamping=10  UpperLimitDampingUnits=N*m/(deg/s)  UpperLimitTransitionRegionWidth=0.1  UpperLimitTransitionRegionWidthUnits=deg  PositionTargetSpecify=on  PositionTargetPriority=Low  PositionTargetValue=-178.55518300385467  PositionTargetValueUnits=deg  VelocityTargetSpecify=off  VelocityTargetPriority=High  VelocityTargetValue=0  VelocityTargetValueUnits=deg/s
  Revolute9 : sm_lib/Joints/Revolute Joint  SenseConstraintForce=off  SenseConstraintForceX=off  SenseConstraintForceY=off  SenseConstraintForceZ=off  SenseConstraintTorque=off  SenseConstraintTorqueX=off  SenseConstraintTorqueY=off  SenseConstraintTorqueZ=off  SenseTotalForce=off  SenseTotalForceX=off  SenseTotalForceY=off  SenseTotalForceZ=off  SenseTotalTorque=off  SenseTotalTorqueX=off  SenseTotalTorqueY=off  SenseTotalTorqueZ=off  CompositeWrenchDir=FollowerOnBase  CompositeWrenchFrame=BaseFrame  EquilibriumPosition=0  EquilibriumPositionUnits=rad  SpringStiffness=0  SpringStiffnessUnits=m*N/rad  DampingCoefficient=0  DampingCoefficientUnits=m*s*N/rad  TorqueActuationMode=NoTorque  MotionActuationMode=ComputedMotion  SensePosition=off  SenseVelocity=off  SenseAcceleration=off  SenseTorqueForce=off  SenseLowerLimitTorqueForce=off  SenseUpperLimitTorqueForce=off  LowerLimitSpecify=off  LowerLimitBound=-90  LowerLimitBoundUnits=deg  LowerLimitStiffness=1e4  LowerLimitStiffnessUnits=N*m/deg  LowerLimitDamping=10  LowerLimitDampingUnits=N*m/(deg/s)  LowerLimitTransitionRegionWidth=0.1  LowerLimitTransitionRegionWidthUnits=deg  UpperLimitSpecify=off  UpperLimitBound=90  UpperLimitBoundUnits=deg  UpperLimitStiffness=1e4  UpperLimitStiffnessUnits=N*m/deg  UpperLimitDamping=10  UpperLimitDampingUnits=N*m/(deg/s)  UpperLimitTransitionRegionWidth=0.1  UpperLimitTransitionRegionWidthUnits=deg  PositionTargetSpecify=off  PositionTargetPriority=High  PositionTargetValue=0  PositionTargetValueUnits=deg  VelocityTargetSpecify=off  VelocityTargetPriority=High  VelocityTargetValue=0  VelocityTargetValueUnits=deg/s
  bras_2_RIGID : Subsystem
  joint_3_RIGID : Subsystem
  joint_4_RIGID : Subsystem
  S1 : PMIOPort  Side=Right
  E1 : PMIOPort  Port=2  Side=Left
  Ref : PMIOPort  Port=3  Side=Left
  Ref1 : PMIOPort  Port=4  Side=Right
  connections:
  Interface1/RConn2 -- Revolute15/RConn2
  Interface1/RConn1 -- Revolute15/LConn2
  Interface1/LConn1 -- E1/RConn1
  Interface1/LConn2 -- Ref/RConn1
  BIELLE_3_RIGID/LConn1 -- Revolute17/RConn1
  Cylindrical1/LConn1 -- joint_3_RIGID/LConn1
  Revolute15/RConn1 -- bras_2_RIGID/LConn1
  Revolute10/RConn1 -- joint_4_RIGID/LConn1
  Revolute17/LConn1 -- joint_3_RIGID/LConn2
  Revolute10/LConn1 -- bras_2_RIGID/RConn1
  S1/RConn1 -- Revolute9/RConn1
  Revolute9/LConn1 -- joint_3_RIGID/RConn1
  BIELLE_3_RIGID/RConn1 -- Revolute18/LConn1
  Revolute15/LConn1 -- Ref1/RConn1
  Revolute18/RConn1 -- joint_4_RIGID/RConn2
  BIELLE_4_RIGID/LConn1 -- Cylindrical1/RConn1
  Revolute19/RConn1 -- joint_4_RIGID/RConn1
  BIELLE_4_RIGID/RConn1 -- Revolute19/LConn1
